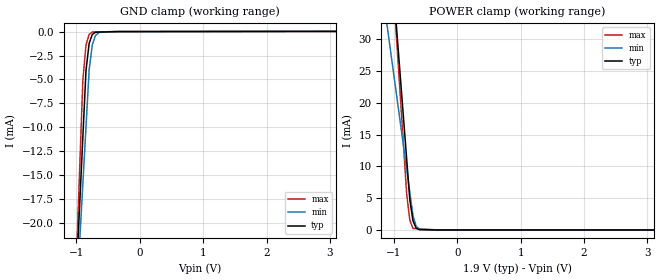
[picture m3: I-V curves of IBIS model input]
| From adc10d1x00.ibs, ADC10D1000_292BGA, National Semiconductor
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[Model] input
Model_type Input
Vinl = 570.000mV
Vinh = 1.33000V
C_comp .915pF .915pF .915pF
| variable typ   min   max
[Voltage Range] 1.90000V 1.80000V 2.00000V
[POWER Clamp Reference] 1.90000V 1.80000V 2.00000V
[GND Clamp Reference] 0.00000V 0.00000V 0.00000V
[Temperature Range]   25   85   -40
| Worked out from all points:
|   GND clamp passes 1 mA (typ) near -0.79 V on its own axis
|   POWER clamp passes 1 mA (typ) near -0.68 V on its own axis
[GND Clamp]
-1.9V     -151.3mA   -135.5mA   -189.6mA
-900mV    -11.06mA   -15.93mA   -5.109mA
-850mV    -4.051mA   -9.95mA    -1.379mA
-800mV    -1.216mA   -3.971mA   -291.9uA
-750mV    -299.9uA   -1.351mA   -48.82uA
-700mV    -63.26uA   -409.8uA   -42.22uA
-650mV    -54.45uA   -124.2uA   -35.62uA
-600mV    -45.63uA   -29.8uA    -29.01uA
-375mV    -5.964uA   -7.653uA   703.9nA
-350mV    -1.556uA   -5.192uA   1.002uA
-300mV    -1.484uA   -270.5nA   1.598uA
3.8V      4.386uA    52.94uA    50.48uA
[POWER Clamp]
-1.9V     153.1mA    90.15mA    174.4mA
-900mV    24.08mA    16.89mA    20.98mA
-800mV    11.18mA    9.559mA    5.64mA
-750mV    4.727mA    5.895mA    1.537mA
-700mV    1.44mA     2.232mA    225.9uA
-650mV    275.4uA    591.4uA    197.6uA
-600mV    44.53uA    127uA      169.4uA
-500mV    29.69uA    76.17uA    112.9uA
-300mV    0A         0A         0A
3.8V      0A         0A         0A
